(* Logix 5000 AddOnInstructionDefinition export AMCI_3202_AOP_Configure; software revision 20.03 *)

ADD_ON_INSTRUCTION AMCI_3202_AOP_Configure   (* revision 1.0 *)
VAR_INPUT
   channel_number : INT; {required}
   capture_input : BOOL; {required}
   capture_input_active_state : BOOL; {required}
   external_input : BOOL; {required}
   external_input_active_state : BOOL; {required}
   home_input : BOOL; {required}
   home_input_active_state : BOOL; {required}
   Emergency_Stop : BOOL; {required}
   Emergency_Stop_active_state : BOOL; {required}
   CW_Limit : BOOL; {required}
   CW_Limit_actitve_state : BOOL; {required}
   CCW_Limit : BOOL; {required}
   CCW_Limit_active_state : BOOL; {required}
   Backplane_Home_Proximity_Enable : BOOL;
   Quad_Encoder : BOOL; {required}
   Diagnostic_Feedback : BOOL;
   _0_CW_CCW_1_step_direction : BOOL; {required}
   _0_enable_1_disable_channel : BOOL;
   Starting_Speed : DINT; {required}
   _0_limit_home_1_marker_pulse_home : BOOL;
END_VAR
VAR_IN_OUT
   AMCI_3202_output_data : AM:1756_3202:O:0; {required}
END_VAR
VAR
   command_data_block : DINT[8];
        [0].31   // Mode Bit 1=Configuraiton Mode 0=Command Mode
END_VAR

ROUTINE Logic   (* ladder *)
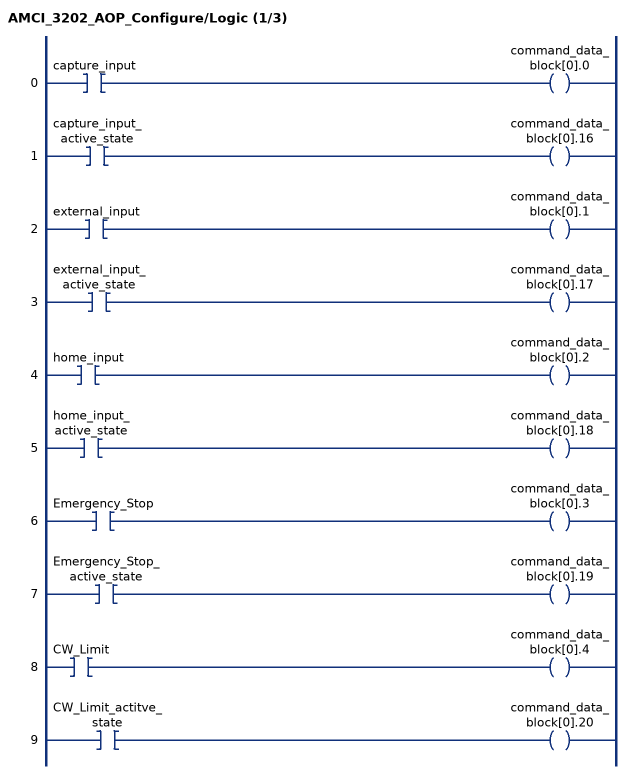
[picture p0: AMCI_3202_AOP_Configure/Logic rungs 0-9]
   0: XIC(capture_input)OTE(command_data_block[0].0);
   1: XIC(capture_input_active_state)OTE(command_data_block[0].16);
   2: XIC(external_input)OTE(command_data_block[0].1);
   3: XIC(external_input_active_state)OTE(command_data_block[0].17);
   4: XIC(home_input)OTE(command_data_block[0].2);
   5: XIC(home_input_active_state)OTE(command_data_block[0].18);
   6: XIC(Emergency_Stop)OTE(command_data_block[0].3);
   7: XIC(Emergency_Stop_active_state)OTE(command_data_block[0].19);
   8: XIC(CW_Limit)OTE(command_data_block[0].4);
   9: XIC(CW_Limit_actitve_state)OTE(command_data_block[0].20);
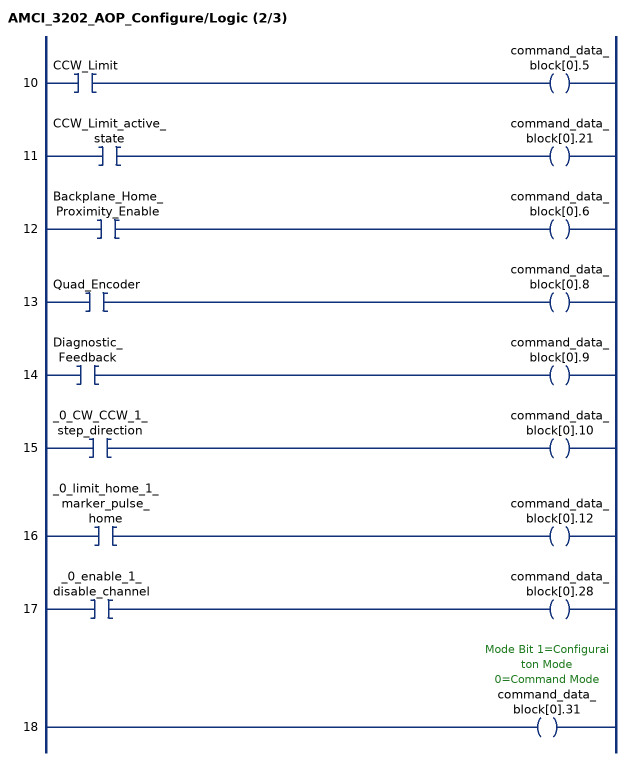
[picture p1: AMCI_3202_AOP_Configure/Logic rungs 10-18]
   10: XIC(CCW_Limit)OTE(command_data_block[0].5);
   11: XIC(CCW_Limit_active_state)OTE(command_data_block[0].21);
   12: XIC(Backplane_Home_Proximity_Enable)OTE(command_data_block[0].6);
   13: XIC(Quad_Encoder)OTE(command_data_block[0].8);
   14: XIC(Diagnostic_Feedback)OTE(command_data_block[0].9);
   15: XIC(_0_CW_CCW_1_step_direction)OTE(command_data_block[0].10);
   16: XIC(_0_limit_home_1_marker_pulse_home)OTE(command_data_block[0].12);
   17: XIC(_0_enable_1_disable_channel)OTE(command_data_block[0].28);
   18: OTE(command_data_block[0].31);
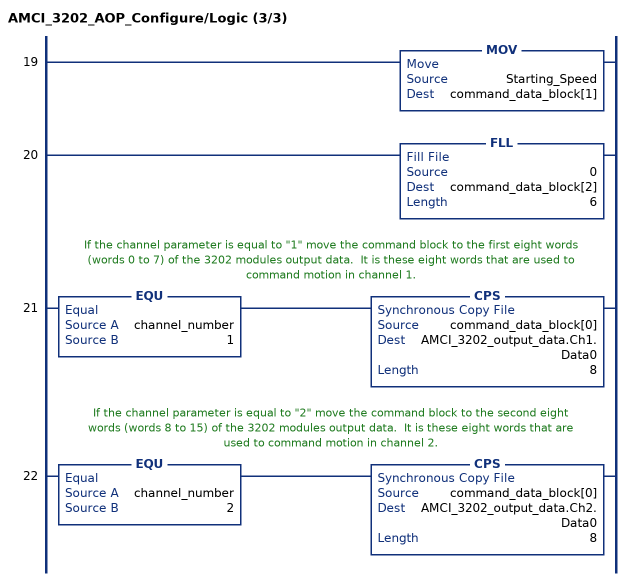
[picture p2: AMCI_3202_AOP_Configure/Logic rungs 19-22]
   19: MOV(Starting_Speed,command_data_block[1]);
   20: FLL(0,command_data_block[2],6);
   // If the channel parameter is equal to "1" move the command block to the first eight words (words 0 to 7) of the 3202 modules output data.  It is these eight words that are used to command motion in channel 1.
   21: EQU(channel_number,1)CPS(command_data_block[0],AMCI_3202_output_data.Ch1.Data0,8);
   // If the channel parameter is equal to "2" move the command block to the second eight words (words 8 to 15) of the 3202 modules output data.  It is these eight words that are used to command motion in channel 2.
   22: EQU(channel_number,2)CPS(command_data_block[0],AMCI_3202_output_data.Ch2.Data0,8);
END_ROUTINE
END_ADD_ON_INSTRUCTION
